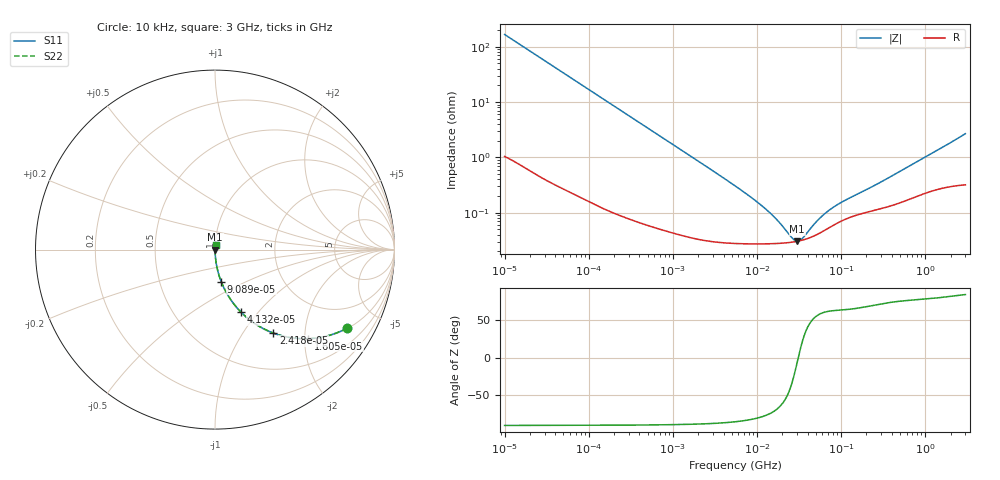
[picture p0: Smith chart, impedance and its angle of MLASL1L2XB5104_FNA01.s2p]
! MLASL1L2XB5104_FNA01  S-PARAMETER MODEL  ( Standard Model )
! Model Generated by TAIYO YUDEN Corporation (http://www.ty-top.com)
! Version 1.0
! TAIYO YUDEN Control No. 220601
! Copyright(c) 2010 TAIYO YUDEN CO.,LTD. All Rights Reserved.
! Product Description (link to TY-COMPAS)
! https://ds.yuden.co.jp/TYCOMPAS/or/detail?pn=MLASL1L2XB5104KFNA01&u=M
! Products Name : Multilayer Ceramic Capacitors
! Characteristics :
!  Capacitance : 0.1 [uF] , Rated Voltage : 10 [V] , TCC : X5R
!  Case Size : 1.0 x 0.5 / 0.039 x 0.02 [mm/inch] , Thickness : 0.2 / 0.008 [mm/inch]
!  (Conditions: Temperature = 25 [degC] , DC Bias Voltage = 0 [V])
! External Node Assignments :
!  1  o---| |---o  2
! GND o---------o GND
! Frequency Range : 10kHz  -  3GHz  [ 401 STEP ]
# MHZ S RI R 50
! Freq[MHz].  S11 Real  S11 Imag  S21 Real  S21 Imag  S12 Real  S12 Imag  S22 Real  S22 Imag
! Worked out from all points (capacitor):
!   401 points, 10 kHz to 3 GHz, reference 50 ohm
!   read as one part in series: C = 95.4 nF near 10.65 kHz
!   lowest |Z| = 30.5 mohm at 30.06 MHz (marker M1)
!   series resonance near 30.96 MHz, so ESL is about 280 pH
!   S11 on the Smith chart (normalised r, x): 10 kHz: 1.02, -3.33; 16.05 kHz: 1.01, -2.08; 24.18 kHz: 1.01, -1.38; 41.32 kHz: 1.01, -0.81; 90.89 kHz: 1.00, -0.37; 3 GHz: 1.01, +0.05
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0.01  0.7337 -0.4389  0.2663 0.4389  0.2663 0.4389  0.7337 -0.4389
0.016047  0.5195 -0.4963  0.4805 0.4963  0.4805 0.4963  0.5195 -0.4963
0.024177  0.3247 -0.4648  0.6753 0.4648  0.6753 0.4648  0.3247 -0.4648
0.03211  0.2154 -0.4075  0.7846 0.4075  0.7846 0.4075  0.2154 -0.4075
0.041322  0.1431 -0.3464  0.8569 0.3464  0.8569 0.3464  0.1431 -0.3464
0.056638  0.0826 -0.2711  0.9174 0.2711  0.9174 0.2711  0.0826 -0.2711
0.082683  0.0413 -0.1946  0.9587 0.1946  0.9587 0.1946  0.0413 -0.1946
0.090886  0.0346 -0.1783  0.9654 0.1783  0.9654 0.1783  0.0346 -0.1783
0.212913  0.00717 -0.0787  0.9928 0.0787  0.9928 0.0787  0.00717 -0.0787
0.683653  0.00112 -0.0248  0.9989 0.0248  0.9989 0.0248  0.00112 -0.0248
5.477226  0.000286 -0.00304  0.9997 0.00304  0.9997 0.00304  0.000286 -0.00304
9.070798  0.000275 -0.00174  0.9997 0.00174  0.9997 0.00174  0.000275 -0.00174
13.24217  0.000274 -0.00106  0.9997 0.00106  0.9997 0.00106  0.000274 -0.00106
18.15044  0.000278 -0.000624  0.9997 0.000624  0.9997 0.000624  0.000278 -0.000624
26.49725  0.000293 -0.000174  0.9997 0.000174  0.9997 0.000174  0.000293 -0.000174
30.05882  0.000303 -3.3e-05  0.9997 3.3e-05  0.9997 3.3e-05  0.000303 -3.3e-05
34.09912  0.000316 0.000107  0.9997 -0.000107  0.9997 -0.000107  0.000316 0.000107
45.28751  0.000366 0.000428  0.9996 -0.000428  0.9996 -0.000428  0.000366 0.000428
60.14696  0.000455 0.000757  0.9995 -0.000757  0.9995 -0.000757  0.000455 0.000757
85.08137  0.000617 0.00116  0.9994 -0.00116  0.9994 -0.00116  0.000617 0.00116
374.4521  0.00132 0.00414  0.9987 -0.00414  0.9987 -0.00414  0.00132 0.00414
3000  0.00387 0.0264  0.9961 -0.0264  0.9961 -0.0264  0.00387 0.0264
